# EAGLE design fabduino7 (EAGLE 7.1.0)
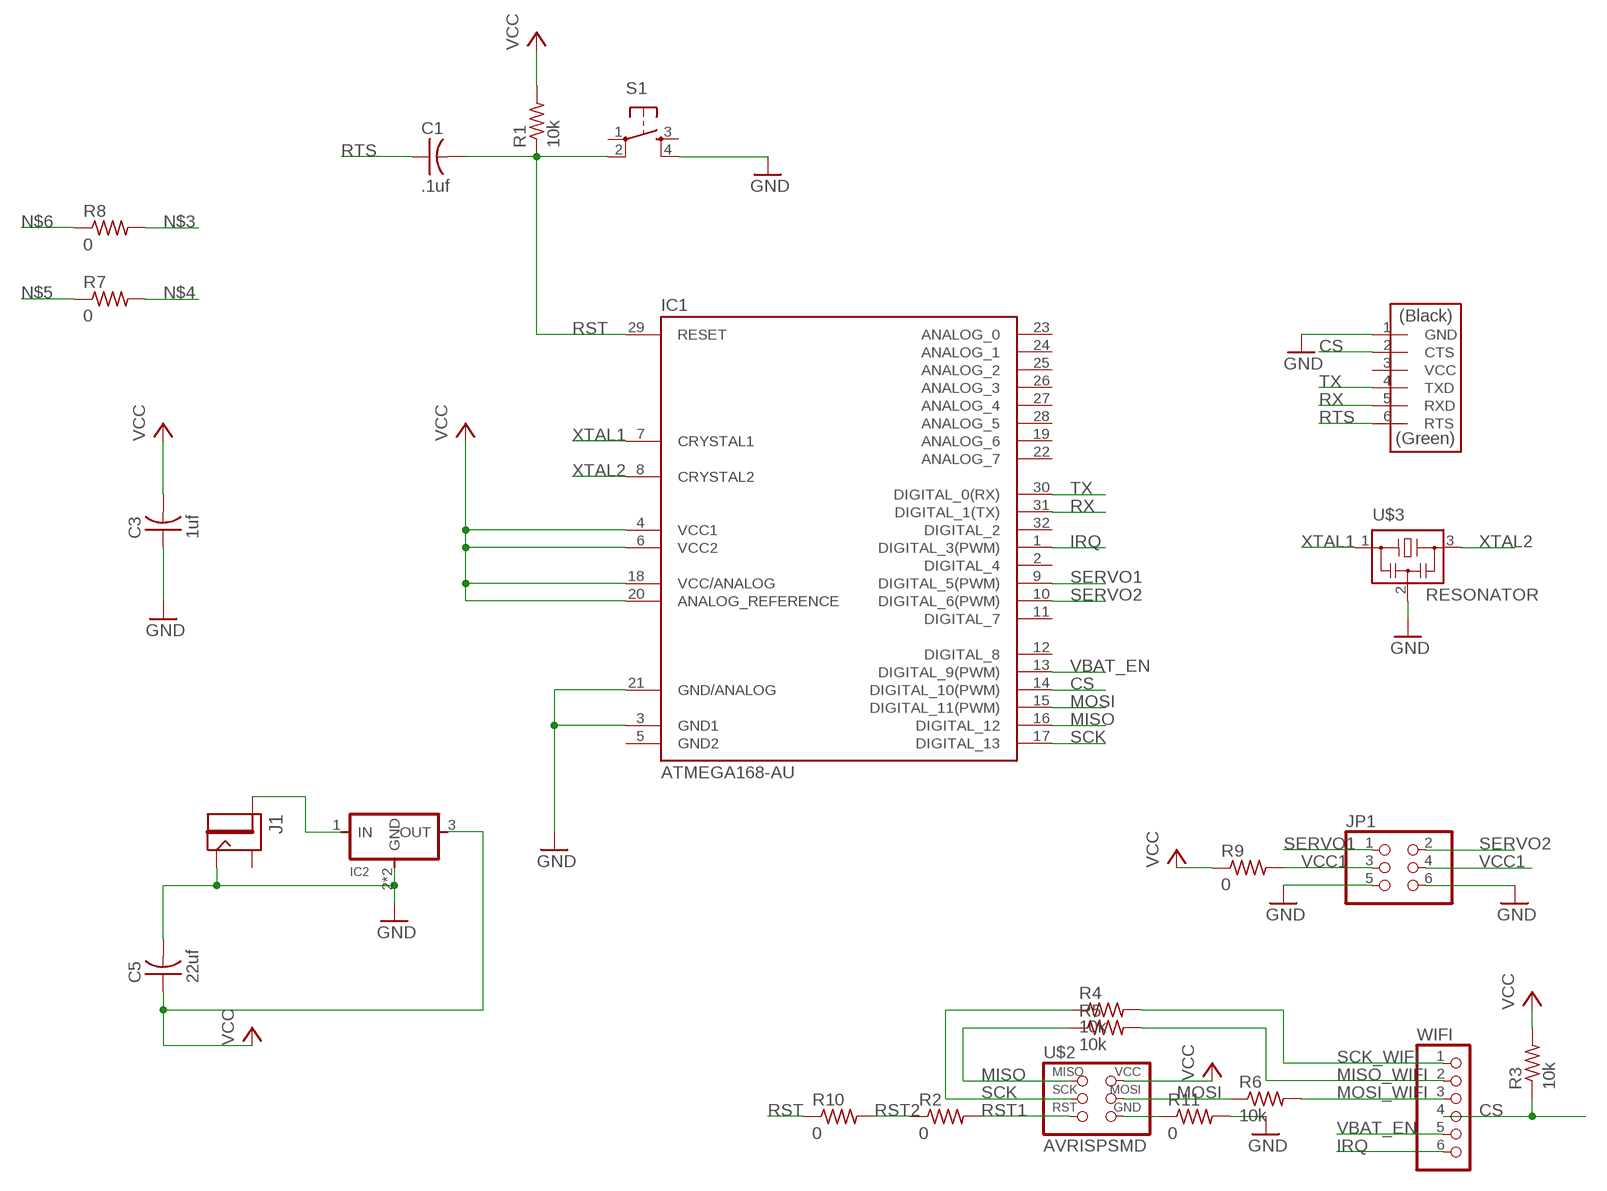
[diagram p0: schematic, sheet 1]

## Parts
C1  .1uf  CAP-US1206  [C1206]
C3  1uf  CAP-US1206  [C1206]
C5  22uf  CAP-US1206  [C1206]
IC1  ATMEGA168-AU  [TQFP32-08]
IC2  REGULATORSOT223  [SOT223]
J1  JACK2.1MM  [JACK_2.1MM]
JP1  PINHD-2X3-SMD  [2X03SMD]
R1  10k  RES-US1206  [R1206]
R2  0  RES-US1206  [R1206]
R3  10k  RES-US1206  [R1206]
R4  10k  RES-US1206  [R1206]
R5  10k  RES-US1206  [R1206]
R6  10k  RES-US1206  [R1206]
R7  0  RES-US1206  [R1206]
R8  0  RES-US1206  [R1206]
R9  0  RES-US1206  [R1206]
R10  0  RES-US1206  [R1206]
R11  0  RES-US1206  [R1206]
S1  6MM_SWITCH6MM_SWITCH  [6MM_SWITCH]
U$1  FTDI-SMD-HEADER  [1X06SMD]
U$2  AVRISPSMD  [2X03SMD]
U$3  RESONATOR  [EFOBM]
WIFI  PINHD-1X6  [1X06]

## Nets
CS: IC1.14(DIGITAL_10(PWM)) R3.1 U$1.2(CTS) WIFI.4
GND: C3.1 C5.2 IC1.3(GND1) IC1.21(GND/ANALOG) IC2.2(GND) IC2.4(GND) J1.CONTACT JP1.5 JP1.6 R11.2 S1.4(S1) U$1.1(GND) U$3.2
IRQ: IC1.1(DIGITAL_3(PWM)) WIFI.6
MISO: IC1.16(DIGITAL_12) R5.1 U$2.1(MISO)
MISO_WIFI: R5.2 WIFI.2
MOSI: IC1.15(DIGITAL_11(PWM)) R6.1 U$2.4(MOSI)
MOSI_WIFI: R6.2 WIFI.3
N$2: IC2.1(IN) J1.PIN
N$3: R8.2
N$4: R7.2
N$5: R7.1
N$6: R8.1
N$7: R11.1 U$2.6(GND)
RST: C1.2 IC1.29(RESET) R1.1 R10.1 S1.2(P1)
RST1: R2.2 U$2.5(RST)
RST2: R2.1 R10.2
RTS: C1.1 U$1.6(RTS)
RX: IC1.31(DIGITAL_1(TX)) U$1.5(RXD)
SCK: IC1.17(DIGITAL_13) R4.1 U$2.3(SCK)
SCK_WIFI: R4.2 WIFI.1
SERVO1: IC1.9(DIGITAL_5(PWM)) JP1.1
SERVO2: IC1.10(DIGITAL_6(PWM)) JP1.2
TX: IC1.30(DIGITAL_0(RX)) U$1.4(TXD)
VBAT_EN: IC1.13(DIGITAL_9(PWM)) WIFI.5
VCC: C3.2 C5.1 IC1.4(VCC1) IC1.6(VCC2) IC1.18(VCC/ANALOG) IC1.20(ANALOG_REFERENCE) IC2.3(OUT) R1.2 R3.2 R9.1 U$2.2(VCC)
VCC1: JP1.3 JP1.4 R9.2
XTAL1: IC1.7(CRYSTAL1) U$3.1
XTAL2: IC1.8(CRYSTAL2) U$3.3
Unconnected: IC1.2(DIGITAL_4) IC1.11(DIGITAL_7) IC1.12(DIGITAL_8) IC1.19(ANALOG_6) IC1.22(ANALOG_7) IC1.23(ANALOG_0) IC1.24(ANALOG_1) IC1.25(ANALOG_2) IC1.26(ANALOG_3) IC1.27(ANALOG_4) IC1.28(ANALOG_5) IC1.32(DIGITAL_2) J1.SHUNT S1.1(P) S1.3(S) U$1.3(VCC)

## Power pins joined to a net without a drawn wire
GND2: IC1.5(GND2)

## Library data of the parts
C1 C3 C5 = fab:CAP-US
IC1 = Arduino-AVR:ATMEGA168
IC2 = fab:REGULATOR
J1 = fab:JACK
JP1 = fab:PINHD-2X3-SMD: PIN HEADER
R1-R11 = fab:RES-US: Resistor (US Symbol)
S1 = fab:6MM_SWITCH: OMRON SWITCH
U$1 = fab:FTDI-SMD-HEADER
U$2 = fab:AVRISP
U$3 = fab:RESONATOR
WIFI = pinhead:PINHD-1X6: PIN HEADER

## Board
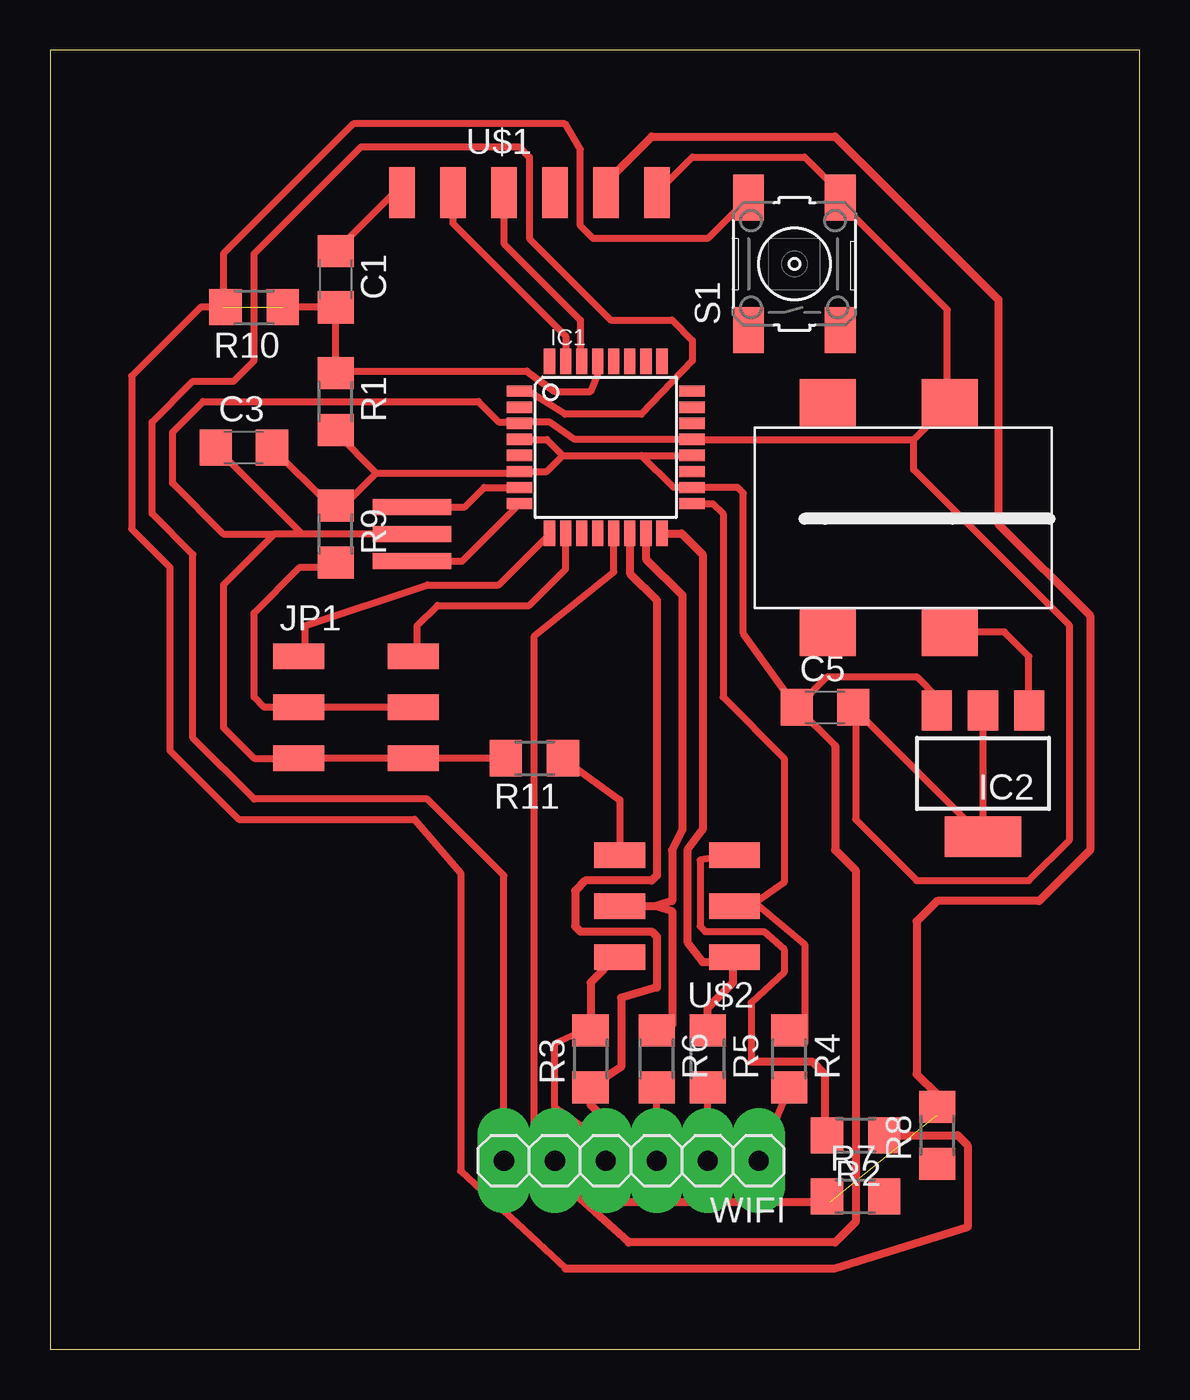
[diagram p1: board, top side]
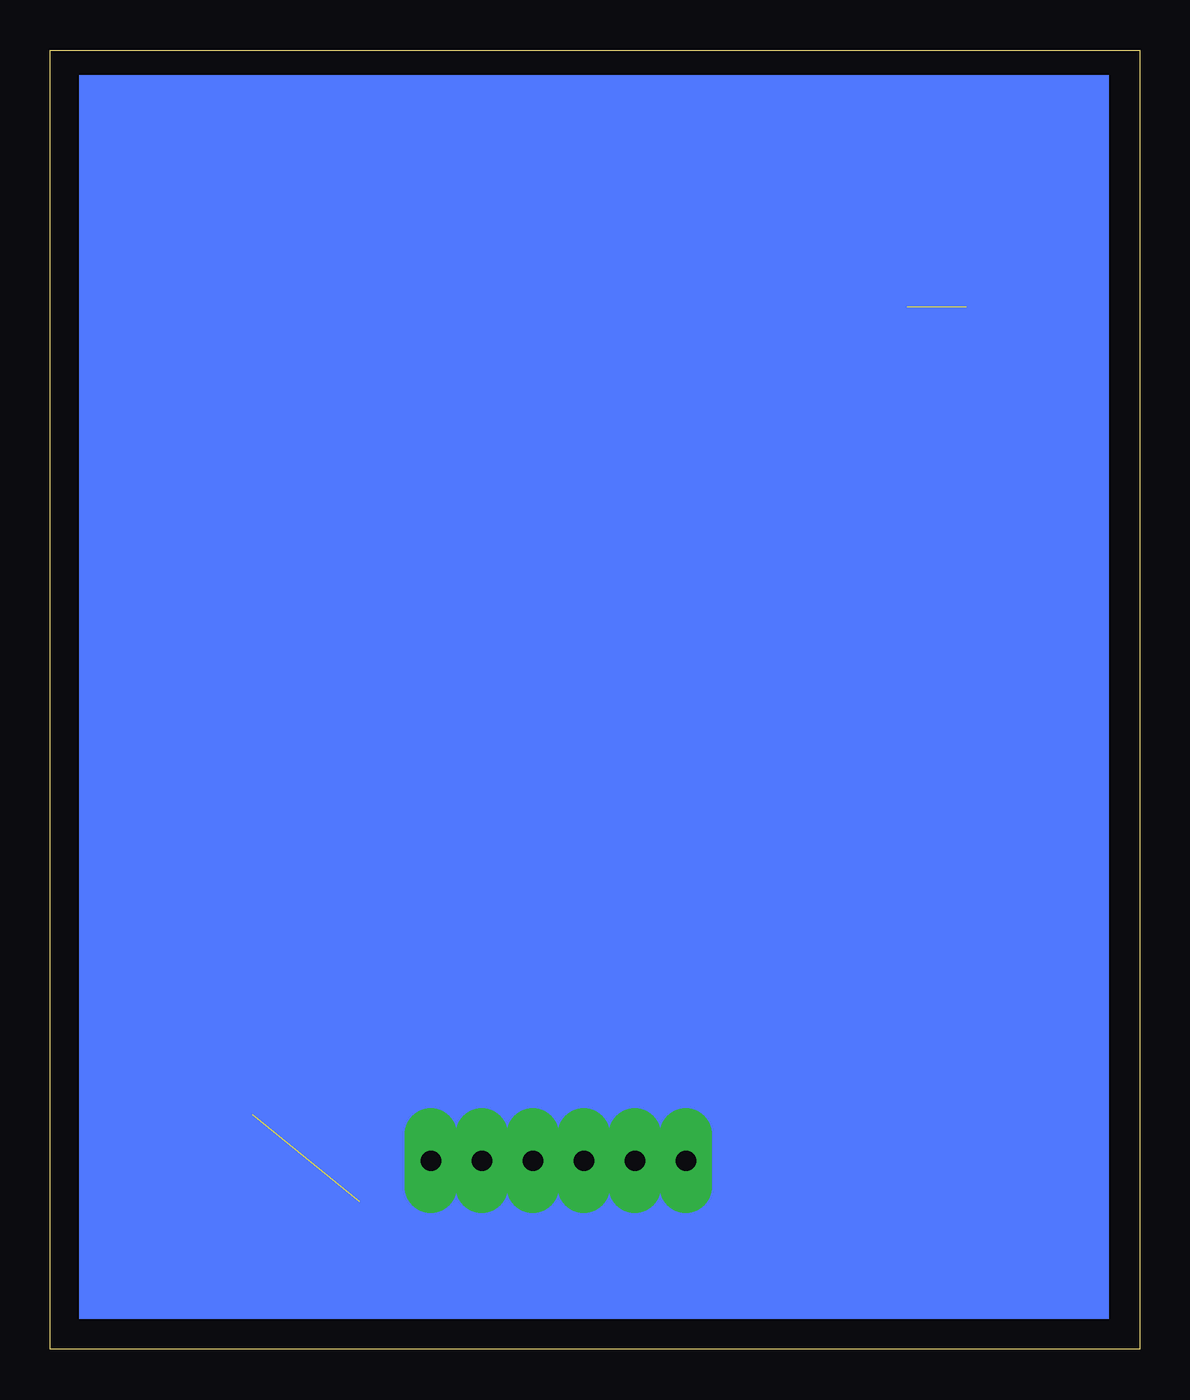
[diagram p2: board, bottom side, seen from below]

Size 54.28 x 64.76 mm. Coordinates in mm from the lower left corner, seen from the top.
Outline: 0,0 54.28,0 54.28,64.76 0,64.76 0,0
Copper layers 16: Bottom 0.035mm
Design rules "fablab": minimum track width 10mil, minimum drill 0.8mm, track to track 16mil, track to pad 16mil, pad to pad 16mil, via to via 16mil, smd to smd 10mil, copper to edge 10mil, drill to drill 10mil, minimum pad ring 0.8mm, minimum via ring 0.8mm, stop-mask expansion 4mil, vias tented up to drill 0mil, thermal gap 1mm

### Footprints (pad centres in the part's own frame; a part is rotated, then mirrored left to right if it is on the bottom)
C1206 = smd 1.6 x 1.8: 1 -1.4,0; 2 1.4,0
TQFP32-08 = smd 1.27 x 0.559: 1 -4.293,2.8; 2 -4.293,2; 3 -4.293,1.2; 4 -4.293,0.4; 5 -4.293,-0.4; 6 -4.293,-1.2; 7 -4.293,-2; 8 -4.293,-2.8; 17 4.293,-2.8; 18 4.293,-2; 19 4.293,-1.2; 20 4.293,-0.4; 21 4.293,0.4; 22 4.293,1.2; 23 4.293,2; 24 4.293,2.8 | smd 0.559 x 1.27: 9 -2.8,-4.293; 10 -2,-4.293; 11 -1.2,-4.293; 12 -0.4,-4.293; 13 0.4,-4.293; 14 1.2,-4.293; 15 2,-4.293; 16 2.8,-4.293; 25 2.8,4.293; 26 2,4.293; 27 1.2,4.293; 28 0.4,4.293; 29 -0.4,4.293; 30 -1.2,4.293; 31 -2,4.293; 32 -2.8,4.293
SOT223 = smd 1.5 x 2: 1 -2.3,-3.15; 2 0,-3.15; 3 2.3,-3.15 | smd 3.8 x 2: 4 0,3.15
JACK_2.1MM = smd 2.388 x 2.794: CONTACT 5.766,-2.413; PIN -5.639,-2.413; PIN1 -5.639,3.683; SHUNT 5.766,3.683
2X03SMD = smd 2.54 x 1.27: 1 -2.857,2.54; 2 2.857,2.54; 3 -2.857,0; 4 2.857,0; 5 -2.857,-2.54; 6 2.857,-2.54
R1206 = smd 1.6 x 1.803: 1 -1.422,0; 2 1.422,0
6MM_SWITCH = smd 2.286 x 1.524: 1 -3.302,2.286; 2 3.302,2.286; 3 -3.302,-2.286; 4 3.302,-2.286
1X06SMD = smd 2.54 x 1.27: 1 0,6.35; 2 0,3.81; 3 0,1.27; 4 0,-1.27; 5 0,-3.81; 6 0,-6.35
EFOBM = smd 0.8 x 3.9: 1 -1.35,0; 2 0,0; 3 1.35,0
1X06 = drill 1.016 long: 1 -6.35,0; 2 -3.81,0; 3 -1.27,0; 4 1.27,0; 5 3.81,0; 6 6.35,0

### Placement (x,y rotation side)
C1  14.22,53.34 270 top
C3  9.65,44.96 0 top
C5  38.61,32 0 top
IC1  27.69,44.96 0 top
IC2  46.48,28.7 180 top
J1  42.42,41.4 90 top
JP1  15.24,32 0 top
R1  14.22,47.24 270 top
R2  40.13,10.67 180 top
R3  26.92,14.48 90 top
R4  36.83,14.48 270 top
R5  32.77,14.48 270 top
R6  30.23,14.48 270 top
R7  40.13,7.62 0 top
R8  44.2,10.67 90 top
R9  14.22,40.64 270 top
R10  10.16,51.94 180 top
R11  24.13,29.46 180 top
S1  37.08,54.1 90 top
U$1  23.88,57.66 270 top
U$2  31.24,22.1 180 top
U$3  18.03,40.64 270 top
WIFI  28.96,9.4 180 top

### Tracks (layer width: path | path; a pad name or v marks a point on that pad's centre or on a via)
CS  (1 unrouted)
  Top 0.406: IC1.14 28.89,38.68 30.23,37.34 30.23,23.62 29.97,23.37 26.67,23.37 26.16,22.86 26.16,21.08 26.42,20.83 29.97,20.83 30.23,20.57 30.23,18.03 28.45,17.53 28.45,14.07 R3.1 26.92,12.19 27.69,11.43 WIFI.4 27.69,8.13 28.45,7.37 38.86,7.37 | U$1.2 27.69,58.17 29.97,60.45 39.12,60.45 47.24,52.32 47.24,41.15 51.82,36.58 51.82,24.89 49.28,22.35 44.2,22.35 43.18,21.34 43.18,13.72 44.2,12.7 44.2,11.68
GND
  Top 0.356: C3.1 12.57,40.64 U$3.2 11.18,40.64 | IC2.4 IC2.2 | IC2.4 46.18,25.86 | U$1.1 32,59.44 37.59,59.44 39.37,57.66 S1.4 39.37,57.15 44.7,51.82 44.7,47.3 J1.CONTACT 43.02,45.36 | 43.02,45.36 IC1.21 26.14,45.36 24.89,46.23 23.46,46.23 IC1.3 23.32,46.23 22.35,46.23 21.34,47.24 7.62,47.24 6.1,45.72 6.1,43.18 8.64,40.64 11.18,40.64 | IC2.4 46.46,25.55 C5.2 40.13,31.88 40.13,26.42 43.18,23.37 48.77,23.37 50.8,25.4 50.8,36.07 43.02,43.85 43.02,45.36 | 11.18,40.64 8.64,38.1 8.64,30.99 10.16,29.46 JP1.5 JP1.6 R11.2
IRQ
  Top 0.356: WIFI.6 22.61,23.62 18.8,27.43 10.16,27.43 7.11,30.48 7.11,39.62 5.08,41.66 5.08,46.23 7.11,48.26 9.14,48.26 10.16,49.28 10.16,54.61 15.49,59.94 23.37,59.94 23.88,59.44 23.88,55.37 27.94,51.31 30.99,51.31 32,50.29 32,49.28 29.46,46.61 25.65,46.61 23.88,47.75 IC1.1
MISO
  Top 0.406: IC1.16 31.47,40.66 32.51,39.62 32.51,25.91 31.75,24.89 31.75,20.32 32.51,19.3 33.84,19.3 U$2.1 34.04,19.49 34.04,18.29 32.77,17.02 R5.1
MISO_WIFI
  Top 0.356: WIFI.2 R5.2
MOSI
  Top 0.406: IC1.15 29.69,39.4 31.5,37.59 31.5,25.91 30.99,24.89 30.99,22.35 30.23,22.1 | U$2.4 30.23,22.1 | 30.23,22.1 30.99,21.84 30.99,16.15 R6.1
MOSI_WIFI
  Top 0.356: WIFI.3 R6.2
N$2
  Top 0.356: IC2.1 48.77,31.87 48.77,34.54 47.55,35.76 J1.PIN
N$7
  Top 0.356: R11.1 28.38,27.39 U$2.6
RST  (1 unrouted)
  Top 0.356: IC1.29 27.29,48.62 26.92,47.75 25.15,47.75 23.75,48.77 14.33,48.77 R1.1 C1.2 R10.1 | S1.2 32.77,55.37 27.05,55.37 26.42,56.01 26.42,59.82 25.65,61.09 15.11,61.09 8.64,54.61 8.64,51.94
RST1
  Top 0.356: U$2.5 32.39,24.38 32.39,21.08 32.64,20.83 35.56,20.83 36.58,19.94 36.58,18.8 34.92,17.27 34.92,14.35
  Top 0.406: 34.92,14.35 37.97,14.35 38.61,13.72 38.61,10.9 R2.2
RST2
  Top 0.356: R10.2 7.49,51.94 4.06,48.51 4.06,40.89 5.97,38.99 5.97,29.84 9.4,26.42 18.16,26.42 20.45,23.75 20.45,8.89 25.68,4.04
  Top 0.406: 25.68,4.04 39.09,4.04 45.72,6.1 45.72,10.16 45.21,10.67 R2.1
RTS
  Top 0.356: C1.1 17.14,57.66 U$1.6
RX
  Top 0.356: U$1.5 20.07,56.13 25.69,50.51 IC1.31
SCK
  Top 0.356: IC1.17 33.03,42.16 33.53,41.66 33.53,32.51 36.58,29.46 36.58,23.27 34.9,22.1 U$2.3 35.31,22.1 37.59,20.19 37.59,15.24 36.93,15.9 R4.1
SCK_WIFI
  Top 0.356: WIFI.1 R4.2
SERVO1
  Top 0.356: JP1.1 12.7,34.86 12.7,36.07 18.8,38.1 22.35,38.1 24.89,40.63 IC1.9
SERVO2
  Top 0.356: JP1.2 18.29,34.73 18.29,36.07 19.3,37.08 23.88,37.08 25.69,38.89 IC1.10
TX
  Top 0.356: U$1.4 22.61,55.12 26.42,51.31 26.42,49.32 IC1.30
VBAT_EN
  Top 0.356: WIFI.5 24.13,10.16 24.13,35.56 28.09,38.75 IC1.13
VCC
  Top 0.356: IC1.4 24.75,45.36 25.55,44.56 | 25.55,44.56 29.46,44.56 | 29.46,44.56 IC1.20 | C3.2 13.95,42.06 R9.1 14.63,42.06 16.26,43.69 | 16.26,43.69 23.32,43.69 IC1.6 24.75,43.76 25.55,44.56 | 29.46,44.56 31.06,42.96 IC1.18 34.26,42.96 34.54,42.67 34.54,35.68 C5.1 | R1.2 14.22,45.72 16.26,43.69 | C5.1 38.73,33.53 43.18,33.53 44.18,32.53 IC2.3 | U$2.2 28.38,19.75 28.45,19.81 | C5.1 39.12,30.1 | 26.42,7.49 26.42,11.18 25.15,12.07 25.15,15.24 26.57,15.9 R3.2
  Top 0.406: U$2.2 28.19,19.56 26.92,18.29 R3.2 | 39.12,30.1 39.12,24.89 40.13,23.88 40.13,6.35 39.12,5.33 28.83,5.33 26.42,7.49
VCC1
  Top 0.356: R9.2 14,38.99 12.45,38.99 10.16,36.7 10.16,32.51 10.67,32 JP1.3 JP1.4
XTAL1
  Top 0.356: U$3.1 20.65,41.99 21.62,42.96 IC1.7
XTAL2
  Top 0.356: U$3.3 20.53,39.29 IC1.8
(copper drawn outside any net)
  shapes: Bottom area x1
